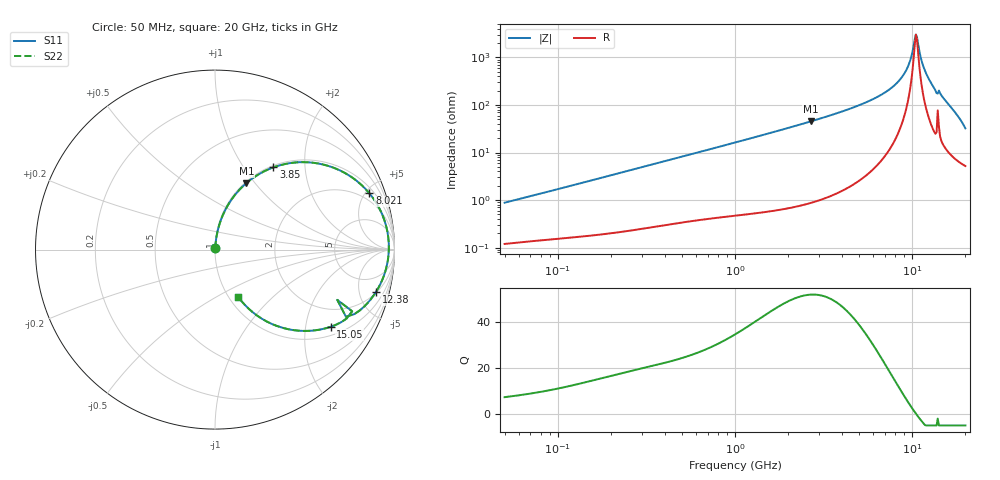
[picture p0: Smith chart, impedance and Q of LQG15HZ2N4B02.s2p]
!Murata Part Number: LQG15HZ2N4B02
!These Parameters are Measured in Series Mode Connection
!  o--[Z]--o
!Port1  Port2
!  o-------o
!Freq. Start=50[MHz] Stop=20[GHz], 401[Steps]
# Hz S RI R 50
!Freq.(Hz) S11(Real) S11(Imag) S21(Real) S21(Imag) S12(Real) S12(Imag) S22(Real) S22(Imag)
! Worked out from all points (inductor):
!   401 points, 50 MHz to 20 GHz, reference 50 ohm
!   read as one part in series: L = 2.74 nH near 51.52 MHz
!   highest Q = 51.9 at 2.687 GHz (marker M1), where L = 2.68 nH
!   self-resonance near 10.5 GHz
!   S11 on the Smith chart (normalised r, x): 50 MHz: 1.00, +0.02; 3.85 GHz: 1.03, +1.38; 8.021 GHz: 1.37, +5.32; 12.38 GHz: 2.11, -7.14; 15.05 GHz: 1.28, -2.76; 20 GHz: 1.10, -0.64
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5e7  0.00127 0.0087  0.9987 -0.0087  0.9987 -0.0087  0.00127 0.0087
1.364002e8  0.00223 0.0228  0.9978 -0.0228  0.9978 -0.0228  0.00223 0.0228
3.721004e8  0.00651 0.0605  0.9935 -0.0605  0.9935 -0.0605  0.00651 0.0605
1e9  0.0299 0.1564  0.9701 -0.1564  0.9701 -0.1564  0.0299 0.1564
2.687447e9  0.175 0.3704  0.825 -0.3704  0.825 -0.3704  0.175 0.3704
2.728004e9  0.1797 0.3744  0.8203 -0.3744  0.8203 -0.3744  0.1797 0.3744
3.850025e9  0.3257 0.4583  0.6743 -0.4583  0.6743 -0.4583  0.3257 0.4583
5.598765e9  0.5762 0.4795  0.4238 -0.4795  0.4238 -0.4795  0.5762 0.4795
7.442007e9  0.8052 0.3699  0.1948 -0.3699  0.1948 -0.3699  0.8052 0.3699
8.020766e9  0.8602 0.3135  0.1398 -0.3135  0.1398 -0.3135  0.8602 0.3135
9.316812e9  0.9445 0.1614  0.0555 -0.1614  0.0555 -0.1614  0.9445 0.1614
9.745021e9  0.9593 0.1059  0.0407 -0.1059  0.0407 -0.1059  0.9593 0.1059
1.034674e10  0.9684 0.0259  0.0316 -0.0259  0.0316 -0.0259  0.9684 0.0259
1.050288e10  0.9685 0.00493  0.0315 -0.00493  0.0315 -0.00493  0.9685 0.00493
1.082228e10  0.9659 -0.0378  0.0341 0.0378  0.0341 0.0378  0.9659 -0.0378
1.131968e10  0.954 -0.1034  0.046 0.1034  0.046 0.1034  0.954 -0.1034
1.166392e10  0.9403 -0.1476  0.0597 0.1476  0.0597 0.1476  0.9403 -0.1476
1.238412e10  0.8974 -0.2353  0.1026 0.2353  0.1026 0.2353  0.8974 -0.2353
1.334722e10  0.8063 -0.3391  0.1937 0.3391  0.1937 0.3391  0.8063 -0.3391
1.504638e10  0.644 -0.4303  0.356 0.4303  0.356 0.4303  0.644 -0.4303
1.721783e10  0.374 -0.435  0.626 0.435  0.626 0.435  0.374 -0.435
2e10  0.1291 -0.2635  0.8709 0.2635  0.8709 0.2635  0.1291 -0.2635
